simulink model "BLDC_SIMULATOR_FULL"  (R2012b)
settings: Solver=ode45  StartTime=0.0  StopTime=0.1  FixedStep=0.0000001  RelTol=1e-6  AbsTol=1e-6
undefined symbols (not defined in the file): CA, Fr, H_Freq, H_Rt, H_Toffon, J, Kd, Ki, Kp, Kv, L, LoopFreq, P, P_Freq, P_Toffon, PAM, PWM, R, Vs
libraries: simulink x4, powerlib_extras x3

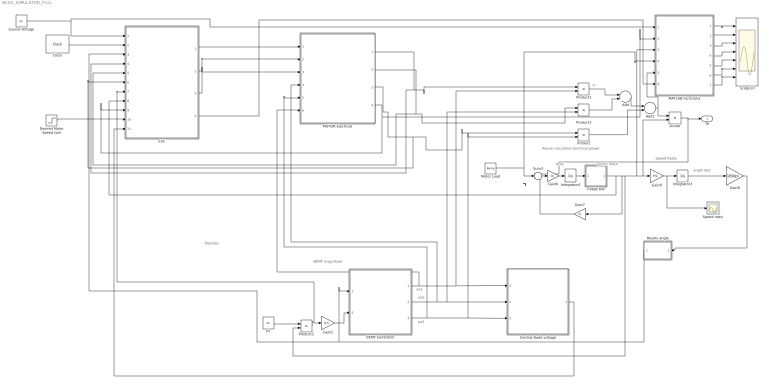
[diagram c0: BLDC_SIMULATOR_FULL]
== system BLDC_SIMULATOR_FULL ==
  note: Above calculates electrical power
  note: ea1
  note: ea2
  note: ea3
  note: vi
  note: Acell
  note: Speed Rad/s
  note: angle elec
  note: BEMF magnitude
  note: Degrees
  note: Tl
  note: speed mech
  Add : Sum
  Add1 : Sum
  BEMF Generator : MATLAB Function  TreatAsAtomicUnit=on
  Central Node voltage : MATLAB Function  TreatAsAtomicUnit=on
  Clock : Clock
  Desired Motor Speed rpm : Step  Time=0.05  Before=4e4  After=2e4  SampleTime=0
  Divide : Product  Inputs=*/
  ESC : Subsystem
  Fudge box : MATLAB Function  TreatAsAtomicUnit=on
  Gain1 : Gain  Gain=0.5
  Gain6 : Gain  Gain=1/J
  Gain7 : Gain  Gain=Fr
  Gain8 : Gain  Gain=180/pi
  Gain9 : Gain  Gain=P/2
  Integrator3 : Integrator
  Integrator4 : Integrator  InitialCondition=0.00001
  Kv : Constant  Value=Kv
  MATLAB Function3 : MATLAB Function  TreatAsAtomicUnit=on
  MOTOR Electrical : Subsystem
  Motor Load : simulink/Sources/Ramp  slope=0  start=0  X0=0
  Product{,1..3} (4 alike) : Product
  Resets angle : MATLAB Function  TreatAsAtomicUnit=on
  Scope10 : Scope  NumInputPorts=7
  Source Voltage : Constant  Value=Vs
  Speed rad/s : Scope
  Sum3 : Sum  Inputs=+--
  Te : Outport
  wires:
  Product1/1 -> Add/1
  Product3/1 -> Add/2
  Add/1 -> Add1/1
  Product/1 -> Add1/2
  Kv/1 -> Product2/1
  Product2/1 -> ESC/7(BEMF), Gain1/1
  BEMF Generator/1(y1) -> MOTOR Electrical/6(ea), Central Node voltage/1(u4), Product1/2
  BEMF Generator/2(y2) -> MOTOR Electrical/4(eb), Product3/2, Central Node voltage/2(u5)
  BEMF Generator/3(y3) -> MOTOR Electrical/5(ec), Product/2, Central Node voltage/3(u6)
  Integrator4/1 -> Fudge box/1(u1)
  Gain6/1 -> Integrator4/1
  Sum3/1 -> Gain6/1
  Gain7/1 -> Sum3/3
  Integrator3/1 -> Gain8/1
  Divide/1 -> Sum3/1, Te/1
  Resets angle/1(yd) -> ESC/3(angle elec), BEMF Generator/1(u1)
  Add1/1 -> Divide/1, MATLAB Function3/5(u5)
  Gain8/1 -> Resets angle/1(ud)
  Gain9/1 -> Speed rad/s/1, Integrator3/1
  MATLAB Function3/1(y1) -> Scope10/1
  MATLAB Function3/2(y2) -> Scope10/2
  MATLAB Function3/3(y3) -> Scope10/3
  MATLAB Function3/4(y4) -> Scope10/4
  MATLAB Function3/5(y5) -> Scope10/5
  MATLAB Function3/6(y6) -> Scope10/6
  MOTOR Electrical/1(Ia) -> ESC/4(Ia), Product1/1
  MOTOR Electrical/3(Ic) -> ESC/6(Ic), Product/1
  MOTOR Electrical/2(Ib) -> ESC/5(Ib), Product3/1
  Source Voltage/1 -> MATLAB Function3/1(u1), ESC/1(V batt)
  Clock/1 -> ESC/2(Clock)
  MOTOR Electrical/4(I-Avg) -> ESC/9(I-AVg), MATLAB Function3/2(u2)
  Gain1/1 -> BEMF Generator/2(u2)
  Desired Motor Speed rpm/1 -> ESC/10(Ref Speed)
  Fudge box/1(y1) -> ESC/8(Speed), MATLAB Function3/3(u3), Divide/2, Gain9/1, Product2/2, Gain7/1
  Central Node voltage/1(y) -> ESC/11(Central node voltage)
  ESC/1(Va) -> MOTOR Electrical/1(In1)
  ESC/2(Vb) -> MOTOR Electrical/2(In2)
  ESC/3(Vc) -> MOTOR Electrical/3(In3)
  MATLAB Function3/7(y7) -> Scope10/7
  ESC/4(ESC losses) -> MATLAB Function3/6(u6)
  Motor Load/1 -> Sum3/2, MATLAB Function3/4(u4)

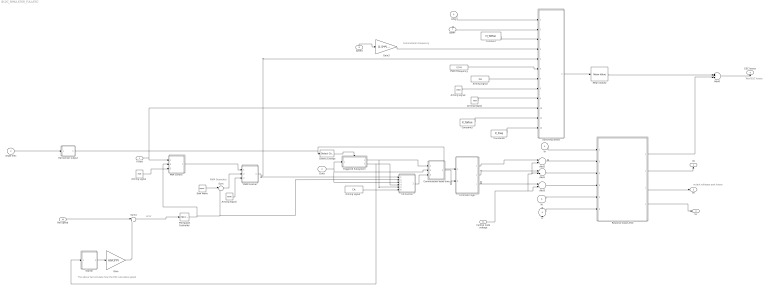
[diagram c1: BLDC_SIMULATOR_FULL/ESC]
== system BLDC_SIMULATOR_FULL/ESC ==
  note: output voltages post losses
  note: Total ESC losses
  note: The above two simulate how the ESC calculates speed
  note: PWM Generator
  note: Commutation Frequency
  note: error
  V batt : Inport
  Clock : Inport  Port=2
  angle elec : Inport  Port=3
  Ia : Inport  Port=4
  Ib : Inport  Port=5
  Ic : Inport  Port=6
  BEMF : Inport  Port=7
  Speed : Inport  Port=8
  I-AVg : Inport  Port=9
  Ref Speed : Inport  Port=10
  Central node voltage : Inport  Port=11
  Add1 : Sum  Inputs=+-
  Add2 : Sum  Inputs=+-
  Add3 : Sum  Inputs=+-
  Add4 : Sum
  Arming Signal : Constant  Value=PWM
  "Arming Signal " : Constant  Value=PAM
  Arming signal : Constant  Value=CA
  "Arming signal " : Constant  Value=PWM
  "Arming signal  " : Constant  Value=PAM
  "Arming signal   " : Constant  Value=CA
  CA Control : MATLAB Function  TreatAsAtomicUnit=on
  Commutation dead time : MATLAB Function  TreatAsAtomicUnit=on
  Constant : Constant  Value=H_Toffon
  Constant5 : Constant  Value=P_Toffon
  Constant8 : Constant  Value=P_Freq
  Controller logic : MATLAB Function  TreatAsAtomicUnit=on
  Detect Change : simulink/Logic and Bit Operations/Detect Change  vinit=64  InputProcessing=Inherited  OutDataTypeStr=boolean
  Gain : Gain  Gain=60/(3*P)
  Gain3 : Gain  Gain=(1.5*P)/pi
  Hall sensor output : MATLAB Function  TreatAsAtomicUnit=on
  Mean Value2 : powerlib_extras/Measurements/Mean Value  Period=1/1000
  "PAM control  " : MATLAB Function  TreatAsAtomicUnit=on
  PID Speed Controller : simulink/Continuous/PID Controller  Controller=PID  TimeDomain=Discrete-time  SampleTime=1/LoopFreq  IntegratorMethod=Trapezoidal  FilterMethod=Forward Euler  Form=Parallel  P=Kp  I=Ki  D=Kd  N=100  InitialConditionSource=internal  InitialConditionForIntegrator=0.4  InitialConditionForFilter=0  ExternalReset=none  LimitOutput=on  UpperSaturationLimit=1  LowerSaturationLimit=0  LinearizeAsGain=off  AntiWindupMode=none  Kb=1  TrackingMode=off  Kt=1  PParamMin=[]  PParamMax=[]  IParamMin=[]  IParamMax=[]  DParamMin=[]  DParamMax=[]  NParamMin=[]  NParamMax=[]  KbParamMin=[]  KbParamMax=[]  KtParamMin=[]  KtParamMax=[]  POutMin=[]  POutMax=[]  IOutMin=[]  IOutMax=[]  DOutMin=[]  DOutMax=[]  NOutMin=[]  NOutMax=[]  KbOutMin=[]  KbOutMax=[]  KtOutMin=[]  KtOutMax=[]  IntegratorOutMin=[]  IntegratorOutMax=[]  FilterOutMin=[]  FilterOutMax=[]  SumOutMin=[]  SumOutMax=[]  SumI1OutMin=[]  SumI1OutMax=[]  SumI2OutMin=[]  SumI2OutMax=[]  SumI3OutMin=[]  SumI3OutMax=[]  SumDOutMin=[]  SumDOutMax=[]  SaturationOutMin=[]  SaturationOutMax=[]  IntegratorContinuousStateAttributes=''  IntegratorStateMustResolveToSignalObject=off  IntegratorRTWStateStorageClass=Auto  FilterContinuousStateAttributes=''  FilterStateMustResolveToSignalObject=off  FilterRTWStateStorageClass=Auto
  PWM Control : MATLAB Function  TreatAsAtomicUnit=on
  PWM FRequency : Constant  Value=H_Freq
  Resistive losses ESC : Subsystem
  Saw Wave : simulink/Sources/Repeating Sequence  rep_seq_t=[0 1/H_Freq]  rep_seq_y=[0 1]
  Starter : MATLAB Function  TreatAsAtomicUnit=on
  Sum : Sum  Inputs=|-+
  Sum4 : Sum  Inputs=|+-
  Switching losses : MATLAB Function  TreatAsAtomicUnit=on
  Triggered Subsystem : Subsystem  TreatAsAtomicUnit=on
  Va : Outport
  Vb : Outport  Port=2
  Vc : Outport  Port=3
  ESC losses : Outport  Port=4
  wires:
  angle elec/1 -> Hall sensor output/1(u1)
  Ia/1 -> Resistive losses ESC/1(Ia)
  Ib/1 -> Resistive losses ESC/5(Ib)
  BEMF/1 -> Switching losses/2(u2)
  Constant/1 -> Switching losses/3(u3)
  Gain3/1 -> Switching losses/4(u4)
  Switching losses/1(y1) -> Mean Value2/1
  Ic/1 -> Resistive losses ESC/6(Ic)
  Resistive losses ESC/1(Ploss-Coduction) -> Add4/2
  Clock/1 -> Commutation dead time/2(u2), CA Control/3(u3), Triggered Subsystem/1(In1)
  I-AVg/1 -> Switching losses/1(u1)
  Arming signal/1 -> Switching losses/7(u7)
  "Arming signal "/1 -> Switching losses/8(u8)
  PWM FRequency/1 -> Switching losses/6(u6)
  Sum4/1 -> PID Speed Controller/1
  Ref Speed/1 -> Sum4/1
  PWM Control/1(y) -> CA Control/1(u1), Switching losses/5(u5)
  Saw Wave/1 -> Sum/1
  Arming Signal/1 -> PWM Control/3(u3)
  Hall sensor output/1(y1) -> Controller logic/1(u1), Detect Change/1
  Detect Change/1 -> Triggered Subsystem/Trigger
  V batt/1 -> Switching losses/10(u10), "PAM control  "/1(u1)
  "PAM control  "/1(y) -> PWM Control/1(u1)
  "Arming signal  "/1 -> "PAM control  "/3(u3)
  "Arming signal   "/1 -> CA Control/6(u6)
  Triggered Subsystem/2(Out2) -> CA Control/4(u4), Starter/1(u1)
  Triggered Subsystem/1(Out1) -> Commutation dead time/1(u1), CA Control/5(u5)
  Starter/1(y) -> Gain/1
  Gain/1 -> Sum4/2
  Speed/1 -> Gain3/1
  "Arming Signal "/1 -> Switching losses/9(u9)
  Constant5/1 -> Switching losses/11(u11)
  Constant8/1 -> Switching losses/12(u12)
  PID Speed Controller/1 -> CA Control/2(u2), Sum/2, "PAM control  "/2(u2)
  Central node voltage/1 -> Add3/2, Add2/2, Add1/2
  Resistive losses ESC/2(Ea) -> Va/1
  Resistive losses ESC/3(Eb) -> Vb/1
  Resistive losses ESC/4(Ec) -> Vc/1
  Add2/1 -> Resistive losses ESC/2(In3)
  Controller logic/1(y1) -> Add2/1
  Controller logic/2(y2) -> Add1/1
  Controller logic/3(y3) -> Add3/1
  Add1/1 -> Resistive losses ESC/3(In4)
  Add3/1 -> Resistive losses ESC/4(In5)
  CA Control/1(y) -> Commutation dead time/3(u3)
  Add4/1 -> ESC losses/1
  Commutation dead time/1(y) -> Controller logic/2(u2)
  Sum/1 -> PWM Control/2(u2)
  Mean Value2/1 -> Add4/1

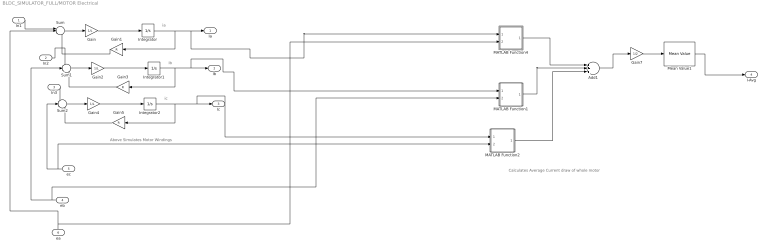
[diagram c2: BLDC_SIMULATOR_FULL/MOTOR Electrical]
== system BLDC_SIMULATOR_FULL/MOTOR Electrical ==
  note: Calculates Average Current draw of whole motor
  note: Above Simulates Motor Windings
  note: i'
  note: ia
  note: i'
  note: ib
  note: i'
  note: ic
  In1 : Inport
  In2 : Inport  Port=2
  In3 : Inport  Port=3
  eb : Inport  Port=4
  ec : Inport  Port=5
  ea : Inport  Port=6
  Add1 : Sum  Inputs=+++
  Gain : Gain  Gain=1/L
  Gain1 : Gain  Gain=R
  Gain2 : Gain  Gain=1/L
  Gain3 : Gain  Gain=R
  Gain4 : Gain  Gain=1/L
  Gain5 : Gain  Gain=R
  Gain7 : Gain  Gain=1/2
  Integrator : Integrator
  Integrator1 : Integrator
  Integrator2 : Integrator
  MATLAB Function1 : MATLAB Function  TreatAsAtomicUnit=on
  MATLAB Function2 : MATLAB Function  TreatAsAtomicUnit=on
  MATLAB Function4 : MATLAB Function  TreatAsAtomicUnit=on
  Mean Value1 : powerlib_extras/Measurements/Mean Value  Period=1/1000
  Sum : Sum  Inputs=+--
  Sum1 : Sum  Inputs=+--
  Sum2 : Sum  Inputs=+--
  Ia : Outport
  Ib : Outport  Port=2
  Ic : Outport  Port=3
  I-Avg : Outport  Port=4
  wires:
  In2/1 -> Sum1/1
  ea/1 -> MATLAB Function4/2(u2), Sum/2
  In1/1 -> Sum/1
  eb/1 -> MATLAB Function1/2(u2), Sum1/2
  ec/1 -> MATLAB Function2/2(u2), Sum2/2
  In3/1 -> Sum2/1
  Sum1/1 -> Gain2/1
  Gain3/1 -> Sum1/3
  Gain/1 -> Integrator/1
  Gain5/1 -> Sum2/3
  Integrator2/1 -> MATLAB Function2/1(u1), Ic/1, Gain5/1
  Sum/1 -> Gain/1
  Integrator/1 -> MATLAB Function4/1(u1), Ia/1, Gain1/1
  Gain4/1 -> Integrator2/1
  Gain1/1 -> Sum/3
  Gain2/1 -> Integrator1/1
  Integrator1/1 -> MATLAB Function1/1(u1), Ib/1, Gain3/1
  Sum2/1 -> Gain4/1
  Add1/1 -> Gain7/1
  Mean Value1/1 -> I-Avg/1
  MATLAB Function2/1(y1) -> Add1/3
  MATLAB Function1/1(y1) -> Add1/2
  MATLAB Function4/1(y1) -> Add1/1
  Gain7/1 -> Mean Value1/1

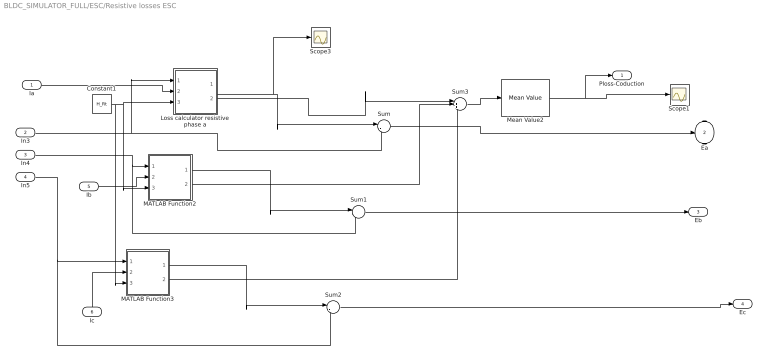
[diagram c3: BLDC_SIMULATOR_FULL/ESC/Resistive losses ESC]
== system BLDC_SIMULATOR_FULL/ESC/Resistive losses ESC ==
  Ia : Inport
  In3 : Inport  Port=2
  In4 : Inport  Port=3
  In5 : Inport  Port=4
  Ib : Inport  Port=5
  Ic : Inport  Port=6
  Constant1 : Constant  Value=H_Rt
  Loss calculator resistive phase a : MATLAB Function  TreatAsAtomicUnit=on
  MATLAB Function2 : MATLAB Function  TreatAsAtomicUnit=on
  MATLAB Function3 : MATLAB Function  TreatAsAtomicUnit=on
  Mean Value2 : powerlib_extras/Measurements/Mean Value  Period=1/500
  Scope1 : Scope
  Scope3 : Scope
  Sum : Sum  Inputs=|-+
  Sum1 : Sum  Inputs=|-+
  Sum2 : Sum  Inputs=|-+
  Sum3 : Sum  Inputs=|+++
  Ploss-Coduction : Outport
  Ea : Outport  Port=2
  Eb : Outport  Port=3
  Ec : Outport  Port=4
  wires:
  Sum2/1 -> Ec/1
  Ic/1 -> MATLAB Function3/2(u2)
  Sum/1 -> Ea/1
  In3/1 -> Sum/2, Loss calculator resistive phase a/1(u1)
  In4/1 -> Sum1/2, MATLAB Function2/1(u1)
  Sum1/1 -> Eb/1
  In5/1 -> MATLAB Function3/1(u1), Sum2/2
  Ia/1 -> Loss calculator resistive phase a/2(u2)
  Ib/1 -> MATLAB Function2/2(u2)
  Loss calculator resistive phase a/1(y1) -> Scope3/1, Sum/1
  Constant1/1 -> MATLAB Function3/3(u3), Loss calculator resistive phase a/3(u3), MATLAB Function2/3(u3)
  MATLAB Function2/1(y1) -> Sum1/1
  MATLAB Function3/1(y1) -> Sum2/1
  Loss calculator resistive phase a/2(y2) -> Sum3/1
  MATLAB Function2/2(y2) -> Sum3/2
  MATLAB Function3/2(y2) -> Sum3/3
  Sum3/1 -> Mean Value2/1
  Mean Value2/1 -> Ploss-Coduction/1, Scope1/1

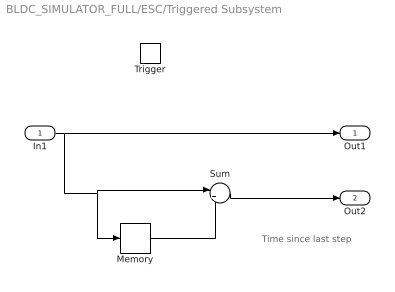
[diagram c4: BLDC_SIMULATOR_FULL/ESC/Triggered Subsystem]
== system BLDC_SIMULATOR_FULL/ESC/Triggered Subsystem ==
  note: Time since last step
  In1 : Inport
  Trigger : TriggerPort
  Memory : Memory  X0=-1  InheritSampleTime=on
  Sum : Sum  Inputs=|+-
  Out1 : Outport
  Out2 : Outport  Port=2
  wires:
  In1/1 -> Out1/1, Memory/1, Sum/1
  Sum/1 -> Out2/1
  Memory/1 -> Sum/2
